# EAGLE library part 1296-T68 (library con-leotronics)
1.27mm SINGLE ROW FEMALE SOCKET Source: http://www.leotronics.co.uk/Conexcon/Data%20Sheets/sec.%20A/1296ing.pdf
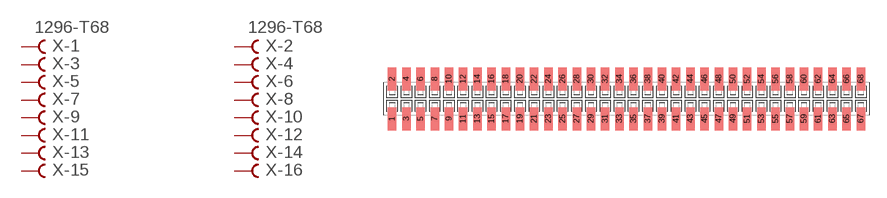
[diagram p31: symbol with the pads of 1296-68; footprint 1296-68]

Designator prefix X; gates -1=FVAL -2=FVAL -3=F -4=F -5=F -6=F -7=F -8=F -9=F -10=F -11=F -12=F -13=F -14=F -15=F -16=F -17=F -18=F -19=F -20=F -21=F -22=F -23=F -24=F -25=F -26=F -27=F -28=F -29=F -30=F -31=F -32=F -33=F -34=F -35=F -36=F -37=F -38=F -39=F -40=F -41=F -42=F -43=F -44=F -45=F -46=F -47=F -48=F -49=F -50=F -51=F -52=F -53=F -54=F -55=F -56=F -57=F -58=F -59=F -60=F -61=F -62=F -63=F -64=F -65=F -66=F -67=F -68=F

## 1296-T68 (OC_FARNELL: unknown; OC_NEWARK: unknown)  [1296-68]
1  -1:B  pas
2  -2:B  pas
3  -3:B  pas
4  -4:B  pas
5  -5:B  pas
6  -6:B  pas
7  -7:B  pas
8  -8:B  pas
9  -9:B  pas
10  -10:B  pas
11  -11:B  pas
12  -12:B  pas
13  -13:B  pas
14  -14:B  pas
15  -15:B  pas
16  -16:B  pas
17  -17:B  pas
18  -18:B  pas
19  -19:B  pas
20  -20:B  pas
21  -21:B  pas
22  -22:B  pas
23  -23:B  pas
24  -24:B  pas
25  -25:B  pas
26  -26:B  pas
27  -27:B  pas
28  -28:B  pas
29  -29:B  pas
30  -30:B  pas
31  -31:B  pas
32  -32:B  pas
33  -33:B  pas
34  -34:B  pas
35  -35:B  pas
36  -36:B  pas
37  -37:B  pas
38  -38:B  pas
39  -39:B  pas
40  -40:B  pas
41  -41:B  pas
42  -42:B  pas
43  -43:B  pas
44  -44:B  pas
45  -45:B  pas
46  -46:B  pas
47  -47:B  pas
48  -48:B  pas
49  -49:B  pas
50  -50:B  pas
51  -51:B  pas
52  -52:B  pas
53  -53:B  pas
54  -54:B  pas
55  -55:B  pas
56  -56:B  pas
57  -57:B  pas
58  -58:B  pas
59  -59:B  pas
60  -60:B  pas
61  -61:B  pas
62  -62:B  pas
63  -63:B  pas
64  -64:B  pas
65  -65:B  pas
66  -66:B  pas
67  -67:B  pas
68  -68:B  pas

## Footprint 1296-68 (pad centres in mm)
1.27mm SINGLE ROW FEMALE SOCKET Source: http://www.leotronics.co.uk/Conexcon/Data%20Sheets/sec.%20A/1296ing.pdf
smd 0.76 x 2.05: 1 -20.955,-1.78; 2 -20.955,1.78; 3 -19.685,-1.78; 4 -19.685,1.78; 5 -18.415,-1.78; 6 -18.415,1.78; 7 -17.145,-1.78; 8 -17.145,1.78; 9 -15.875,-1.78; 10 -15.875,1.78; 11 -14.605,-1.78; 12 -14.605,1.78; 13 -13.335,-1.78; 14 -13.335,1.78; 15 -12.065,-1.78; 16 -12.065,1.78; 17 -10.795,-1.78; 18 -10.795,1.78; 19 -9.525,-1.78; 20 -9.525,1.78; 21 -8.255,-1.78; 22 -8.255,1.78; 23 -6.985,-1.78; 24 -6.985,1.78; 25 -5.715,-1.78; 26 -5.715,1.78; 27 -4.445,-1.78; 28 -4.445,1.78; 29 -3.175,-1.78; 30 -3.175,1.78; 31 -1.905,-1.78; 32 -1.905,1.78; 33 -0.635,-1.78; 34 -0.635,1.78; 35 0.635,-1.78; 36 0.635,1.78; 37 1.905,-1.78; 38 1.905,1.78; 39 3.175,-1.78; 40 3.175,1.78; 41 4.445,-1.78; 42 4.445,1.78; 43 5.715,-1.78; 44 5.715,1.78; 45 6.985,-1.78; 46 6.985,1.78; 47 8.255,-1.78; 48 8.255,1.78; 49 9.525,-1.78; 50 9.525,1.78; 51 10.795,-1.78; 52 10.795,1.78; 53 12.065,-1.78; 54 12.065,1.78; 55 13.335,-1.78; 56 13.335,1.78; 57 14.605,-1.78; 58 14.605,1.78; 59 15.875,-1.78; 60 15.875,1.78; 61 17.145,-1.78; 62 17.145,1.78; 63 18.415,-1.78; 64 18.415,1.78; 65 19.685,-1.78; 66 19.685,1.78; 67 20.955,-1.78; 68 20.955,1.78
